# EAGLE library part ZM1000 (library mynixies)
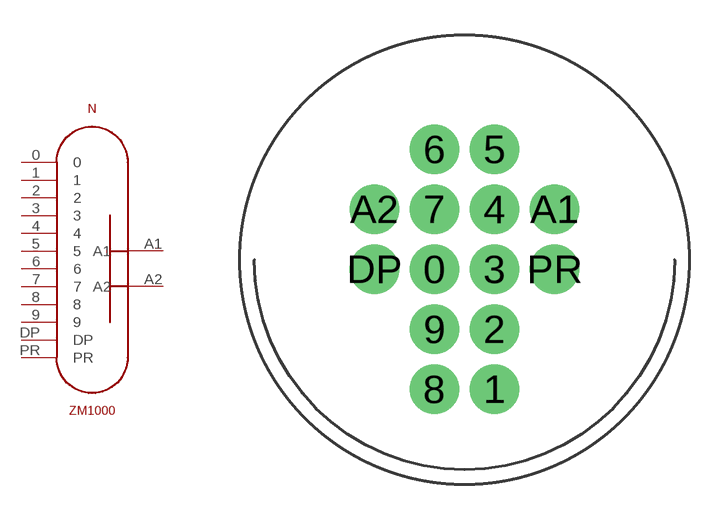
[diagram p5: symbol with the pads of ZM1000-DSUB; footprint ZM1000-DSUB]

Designator prefix N

## ZM1000D-SUB  [ZM1000-DSUB]
0  0  pas
1  1  pas
2  2  pas
3  3  pas
4  4  pas
5  5  pas
6  6  pas
7  7  pas
8  8  pas
9  9  pas
A1  A1  pas
A2  A2  pas
DP  DP  pas
PR  PR  pas

## Footprint ZM1000-DSUB (pad centres in mm)
drill 1.4: 0 -1.27,-0.4; 1 1.27,-5.48; 2 1.27,-2.94; 3 1.27,-0.4; 4 1.27,2.14; 5 1.27,4.68; 6 -1.27,4.68; 7 -1.27,2.14; 8 -1.27,-5.48; 9 -1.27,-2.94; A1 3.81,2.14; A2 -3.81,2.14; DP -3.81,-0.4; PR 3.81,-0.4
